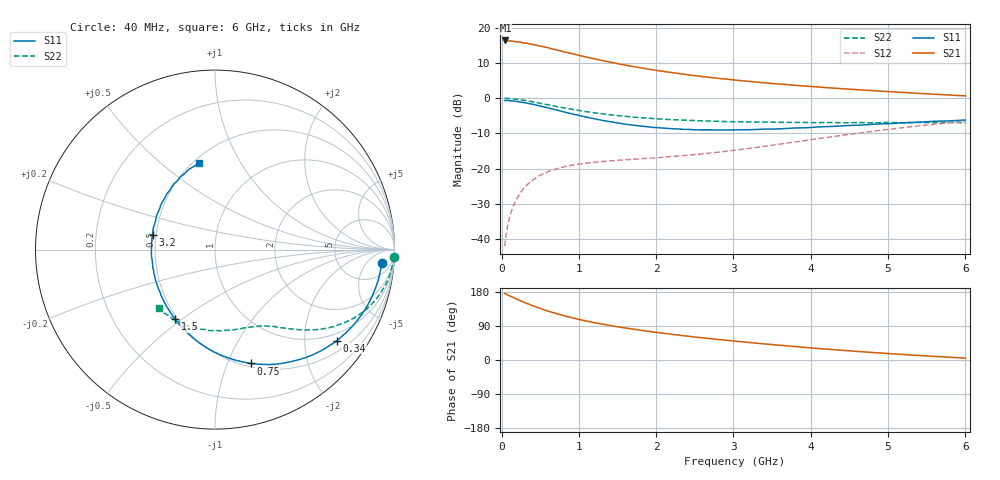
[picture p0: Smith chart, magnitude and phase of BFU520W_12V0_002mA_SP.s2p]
! Filename:  P:\Prog\Test\Noise\ATS_data\Testdata_Net\Run2\BFU520W_APM2013_06_A05_12p0V_002mA_SP_CM01_D.s2p
! Date/Time: Tue 26/Mar/2013 18:01:43
! BFU520W_APM2013_06_A05_12p0V_1to20mA_SP_CM01_Bias2_R.s2p
! MDIF S-parameter v. bias file
! BFU520W_APM2013_06_A05_12p0V_1to20mA_SP_CM01
! Date/time Thu Mar 21 16:35:01 2013
! VAR V_out= 12.0000
! VAR I_out= 2.0000
! VAR V_in= 0.8022
! VAR I_in= 0.0190
! Device data file deembeded for feedlines and parallel
! Original file: \Run2\BFU520W_APM2013_06_A05_12p0V_002mA_SP_CM01_R.s2p
! Feed-files: PR019V01_070313_Feed1.s2p, PR019V01_070313_Feed2.s2p
! Parallel-file: PR019V01_070313_Par.s2p
# MHz S MA R 50
!  Freq-MHz  S11-mag  S11-arg  S21-mag  S21-arg  S12-mag  S12-arg  S22-mag  S22-arg
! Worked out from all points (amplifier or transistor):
!   98 points, 40 MHz to 6 GHz, reference 50 ohm
!   highest |S21| = 16.4 dB at 50 MHz (marker M1)
!   |S21| within 3 dB of that: start of sweep to 768.4 MHz
!   unconditionally stable (mu >= 1): 2.414 GHz to 3.497 GHz
!   at 300 MHz: K = 0.18, MSG = 20.5 dB, |S12| = -25.3 dB
!   at 1.6 GHz: K = 0.78, MSG = 13.5 dB, |S12| = -17.5 dB
!   at 6 GHz: K = 0.82, MSG = 3.6 dB, |S12| = -6.5 dB
!   S11 on the Smith chart (normalised r, x): 40 MHz: 13, -14; 340 MHz: 0.78, -2.82; 750 MHz: 0.53, -1.21; 1.5 GHz: 0.49, -0.47; 3.2 GHz: 0.48, +0.09; 6 GHz: 0.53, +0.68
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40  0.9314 -4.5  6.603 176.0  0.007921 86.2  0.9962 -2.4
50  0.9297 -5.6  6.621 174.8  0.009798 85.7  0.9963 -3.2
90  0.9258 -10.1  6.49 170.8  0.01754 83.2  0.9904 -5.8
120  0.9196 -13.5  6.528 167.9  0.02323 81.4  0.9859 -7.7
220  0.8929 -24.3  6.317 158.7  0.0412 75.1  0.9588 -13.7
340  0.8479 -36.7  6.012 148.3  0.06012 68.2  0.9154 -20.3
420  0.8125 -44.4  5.768 142.0  0.07106 64.3  0.883 -24.1
550  0.7515 -56.4  5.37 132.6  0.08563 58.7  0.8273 -29.5
600  0.7297 -60.8  5.229 129.2  0.09047 56.9  0.8071 -31.3
750  0.6646 -72.7  4.737 120.1  0.1022 52.3  0.7502 -36.0
900  0.6046 -83.7  4.33 112.1  0.1114 49.0  0.7012 -39.6
1050  0.5544 -93.8  3.953 105.0  0.1178 46.6  0.6567 -42.9
1250  0.4978 -106.1  3.529 96.7  0.1249 44.5  0.612 -46.2
1500  0.4461 -120.1  3.102 87.8  0.1313 43.6  0.568 -50.0
1800  0.4026 -135.5  2.708 78.5  0.1381 44.3  0.5293 -53.7
2050  0.3797 -147.3  2.445 71.7  0.1442 45.7  0.5073 -56.9
2500  0.3567 -167.1  2.097 60.7  0.1585 49.1  0.4819 -62.9
3100  0.3566 170.4  1.776 48.2  0.1877 54.3  0.4633 -72.0
3200  0.3572 167.0  1.735 46.3  0.1941 54.9  0.4604 -73.5
4100  0.3911 140.8  1.444 30.4  0.2671 57.0  0.45 -90.3
5200  0.4485 115.5  1.207 14.4  0.3833 51.0  0.4479 -114.2
6000  0.4912 100.5  1.08 4.9  0.4716 43.3  0.4501 -134.1
